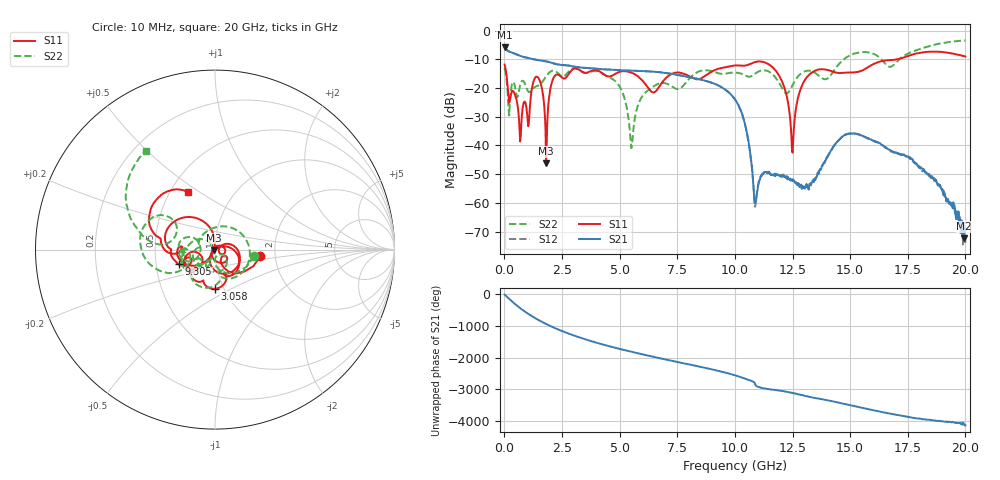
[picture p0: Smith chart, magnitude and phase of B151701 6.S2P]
!  2-Port S-parameters saved by WinCal
! VAR MeasName=S-Parameters (CALIBRATED_DATA) read from VNA (N5244A)
! VAR MeasDate=2015-12-24 19:08:50
! VAR NAME=B151701 6
! VAR FILENAME=B151701 6.S2P
! VAR DATE=2015-12-24 19:08:50
! VAR PHYS_PORTS=1,3
# Hz S DB R 50
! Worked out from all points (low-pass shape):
!   801 points, 10 MHz to 20 GHz, reference 50 ohm
!   highest |S21| = -5.81 dB at 10 MHz (marker M1); lowest = -72.3 dB at 19.95 GHz (marker M2)
!   |S21| within 3 dB of the highest: start of sweep to 679 MHz
!   lowest |S11| = -46.2 dB at 1.809 GHz (marker M3), VSWR 1.01, Z = 49.6 - j0.22 ohm
!   |S11| at or under -10 dB: start of sweep to 17.06 GHz
!   |S22| runs from -40.9 to -3.5 dB; largest |S21 - S12| = 0.0015
!   S11 on the Smith chart (normalised r, x): 10 MHz: 1.67, -0.12; 3.058 GHz: 0.91, -0.42; 9.305 GHz: 0.66, -0.11; 20 GHz: 0.61, +0.45
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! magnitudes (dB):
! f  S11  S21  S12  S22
! 10 MHz  -11.8  -5.8  -5.8  -13.2
! 209.9 MHz  -25.2  -7.3  -7.3  -29.6
! 684.7 MHz  -38.6  -8.8  -8.8  -19.0
! 1.459 GHz  -16.3  -10.3  -10.3  -19.2
! 1.809 GHz  -46.2  -10.7  -10.7  -16.0
! 2.159 GHz  -16.1  -11.5  -11.5  -14.0
! 3.058 GHz  -13.2  -12.6  -12.6  -13.1
! 3.358 GHz  -14.3  -12.9  -12.9  -14.3
! 4.908 GHz  -14.7  -13.8  -13.7  -18.4
! 5.507 GHz  -14.6  -14.0  -14.0  -40.9
! 6.682 GHz  -20.0  -14.5  -14.5  -18.5
! 9.305 GHz  -13.2  -19.2  -19.2  -14.9
! 10.01 GHz  -12.2  -24.0  -24.0  -14.6
! 10.48 GHz  -12.2  -34.0  -34.1  -15.8
! 10.9 GHz  -10.9  -59.7  -60.2  -14.9
! 11.98 GHz  -16.6  -50.5  -50.5  -19.1
! 12.5 GHz  -42.5  -52.4  -52.0  -18.9
! 13.35 GHz  -14.6  -52.8  -53.1  -14.2
! 14.83 GHz  -14.6  -36.2  -36.1  -9.4
! 16.68 GHz  -10.3  -41.4  -41.4  -12.6
! 19.95 GHz  -8.9  -72.3  -69.4  -3.5
! 20 GHz  -9.0  -68.6  -74.3  -3.5
